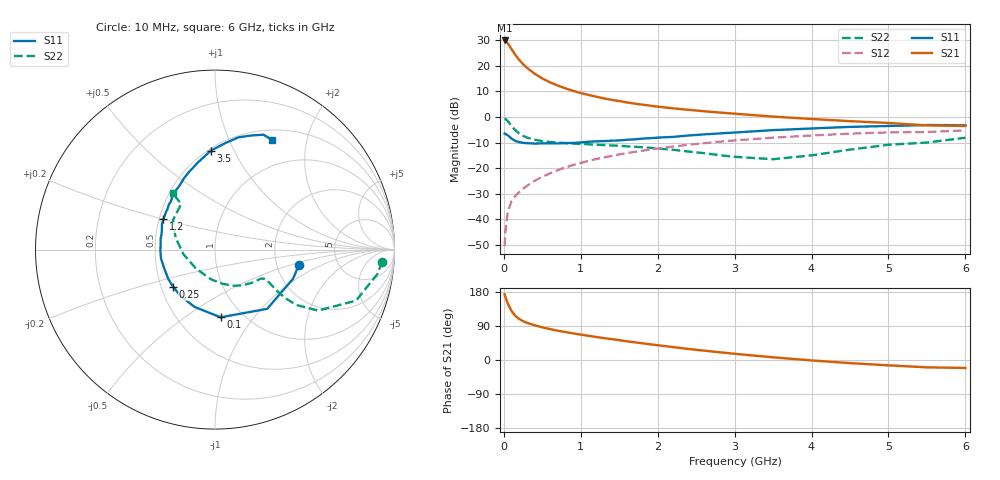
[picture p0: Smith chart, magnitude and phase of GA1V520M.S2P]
! Infineon Technologies  Discrete & RF Semiconductors
! BF775
! Si NPN RF Bipolar Junction Transistor in SOT23
! VCE = 1.5 V  IC = 20 mA
! Common Emitter S-Parameters:  May  1996
# GHz  S  MA  R  50
!  f  S11  S21  S12  S22
! GHz  MAG  ANG  MAG  ANG  MAG  ANG  MAG  ANG
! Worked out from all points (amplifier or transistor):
!   36 points, 10 MHz to 6 GHz, reference 50 ohm
!   highest |S21| = 29.9 dB at 10 MHz (marker M1)
!   |S21| within 3 dB of that: start of sweep to 91.99 MHz
!   unconditionally stable (mu >= 1): 286.2 MHz to end of sweep
!   at 250 MHz: K = 0.96, MSG = 24.3 dB, |S12| = -28.0 dB
!   at 1.4 GHz: K = 1.18, MAG = 8.4 dB, |S12| = -15.2 dB
!   at 6 GHz: K = 1.03, MAG = -0.2 dB, |S12| = -5.3 dB
!   S11 on the Smith chart (normalised r, x): 10 MHz: 2.65, -0.60; 100 MHz: 0.79, -0.70; 250 MHz: 0.58, -0.27; 1.2 GHz: 0.53, +0.20; 3.5 GHz: 0.52, +0.82; 6 GHz: 0.63, +1.46
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0.01  0.4744 -10.6  31.1 173.3  0.003 90.4  0.9346 -4.1
0.02  0.464 -20.5  30.45 166.7  0.0057 82.7  0.9137 -8.7
0.05  0.4399 -48.6  27.54 149.6  0.0135 73.1  0.8354 -19.9
0.1  0.3784 -85.2  21.1 129.4  0.0228 66.5  0.6671 -30.6
0.15  0.3393 -109.4  16.24 116.4  0.0288 63.1  0.5491 -34.2
0.2  0.3225 -126.5  12.98 108.3  0.0341 63.9  0.4761 -34.6
0.25  0.312 -138.2  10.69 102.4  0.0396 64.5  0.427 -33.9
0.3  0.3078 -147.6  9.099 98.1  0.0452 66.2  0.3967 -33.1
0.4  0.3015 -161.7  6.987 91.7  0.0564 67.6  0.3598 -31.6
0.5  0.3052 -171.1  5.63 86.1  0.0678 68.5  0.3373 -30.6
0.6  0.3044 -178.8  4.736 81.6  0.0794 68.5  0.3251 -30.4
0.8  0.3087 168.9  3.615 73.8  0.1032 68.1  0.3084 -31.6
0.9  0.3101 163.7  3.229 70.3  0.1152 67.4  0.3019 -32.4
1.1  0.3279 154.5  2.688 63.9  0.1387 65.8  0.2927 -35.6
1.2  0.3339 149.7  2.485 60.7  0.1502 64.8  0.2865 -37.2
1.6  0.3587 136.0  1.92 49.3  0.1965 60.4  0.2666 -45.4
2.2  0.4075 119.0  1.472 34.1  0.2641 52.7  0.2284 -61.8
2.8  0.476 104.3  1.219 20.5  0.3282 44.4  0.1792 -86.6
3.5  0.5522 92.3  1.015 7.0  0.3936 34.1  0.1495 -134.8
4.5  0.639 78.2  0.827 -8.2  0.4714 19.8  0.2304 162.7
5.5  0.695 67.1  0.683 -19.4  0.5069 5.4  0.3161 126.6
6  0.6888 62.3  0.666 -21.0  0.5457 1.2  0.3933 126.8
